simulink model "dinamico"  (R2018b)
settings: Solver=VariableStepAuto  StartTime=0.0  StopTime=10  RelTol=1e-3
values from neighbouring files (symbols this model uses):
  o = 1.5    [dati_simu.m]
  s = 300e-3    (= 0.3)    [dati_simu.m]
  tau = 1/(2*pi*fband)    (= 9.94718394324e-05)    [dati_simu.m]

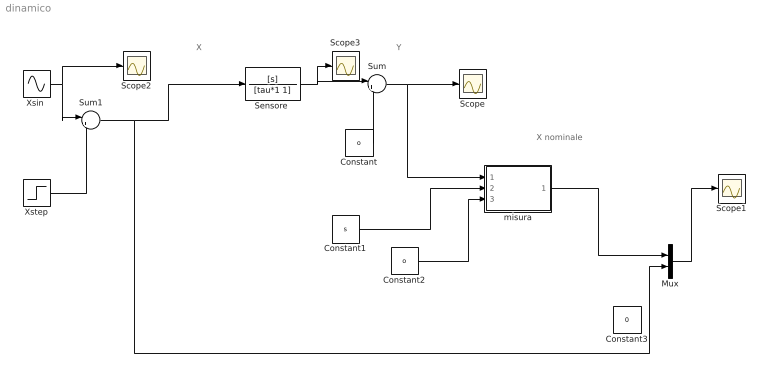
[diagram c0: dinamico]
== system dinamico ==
  note: X
  note: Y
  note: X nominale
  Constant : Constant  Value=o
  Constant1 : Constant  Value=s
  Constant2 : Constant  Value=o
  Constant3 : Constant  Commented=on  Value=0
  Mux : Mux  Inputs=2
  Scope{,1..3} (4 alike) : Scope
  "Sensore " : TransferFcn  Numerator=[s]  Denominator=[tau*1 1]
  Sum : Sum  Inputs=|++
  Sum1 : Sum  Inputs=|++
  "Xsin " : Sin  Frequency=1600*2*pi  Samples=100  SampleTime=0
  Xstep : Step  After=0  SampleTime=0
  misura : MATLAB Function  TreatAsAtomicUnit=on
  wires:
  "Sensore "/1 -> Scope3/1, Sum/1
  Sum/1 -> misura/1(y), Scope/1
  Constant/1 -> Sum/2
  Constant1/1 -> misura/2(s)
  Constant2/1 -> misura/3(o)
  misura/1(xn) -> Mux/1
  Mux/1 -> Scope1/1
  "Xsin "/1 -> Sum1/1, Scope2/1
  Xstep/1 -> Sum1/2
  Sum1/1 -> Mux/2, "Sensore "/1

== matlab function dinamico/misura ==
function xn = fcn(y,s,o) %xnominale


xn = (y-o)/s;
